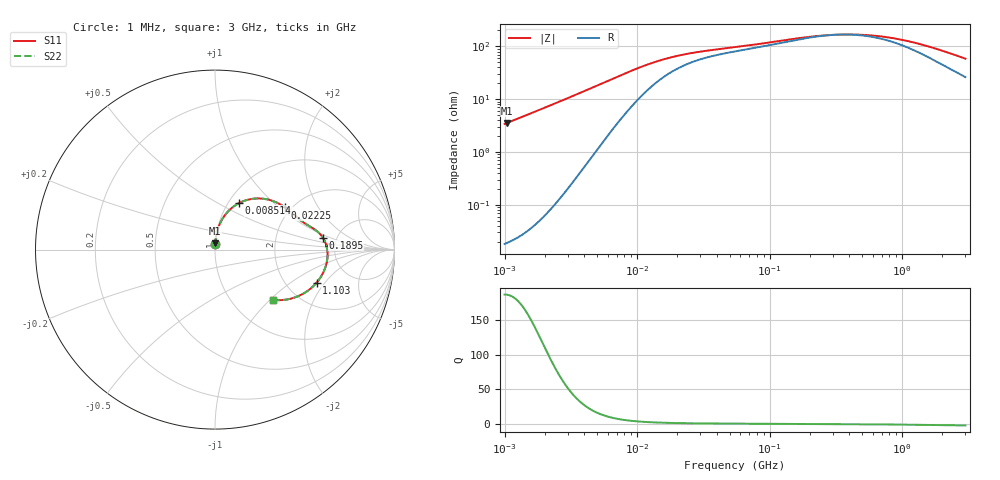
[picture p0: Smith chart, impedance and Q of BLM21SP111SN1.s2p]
! BLM21SP111SN1
# Hz S RI R 50
!Freq.(Hz) S11(Real) S11(Imag) S21(Real) S21(Imag) S12(Real) S12(Imag) S22(Real) S22(Imag)
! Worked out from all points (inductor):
!   401 points, 1 MHz to 3 GHz, reference 50 ohm
!   read as one part in series: L = 543 nH near 1.041 MHz
!   highest Q = 187 at 1.041 MHz (marker M1), where L = 541 nH
!   self-resonance near 332.2 MHz
!   S11 on the Smith chart (normalised r, x): 1 MHz: 1.00, +0.07; 8.514 MHz: 1.12, +0.64; 22.25 MHz: 1.86, +1.10; 189.5 MHz: 3.87, +0.81; 1.103 GHz: 2.90, -1.66; 3 GHz: 1.53, -1.05
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1000000  0.00134 0.0339  0.9987 -0.0339  0.9987 -0.0339  0.00134 0.0339
1040844  0.00144 0.0353  0.9986 -0.0353  0.9986 -0.0353  0.00144 0.0353
2139570  0.00613 0.0732  0.9939 -0.0732  0.9939 -0.0732  0.00613 0.0732
3823119  0.0223 0.1322  0.9777 -0.1322  0.9777 -0.1322  0.0223 0.1322
5938264  0.0625 0.2012  0.9375 -0.2012  0.9375 -0.2012  0.0625 0.2012
8513927  0.1352 0.2598  0.8648 -0.2598  0.8648 -0.2598  0.1352 0.2598
1.126754e7  0.2167 0.2838  0.7833 -0.2838  0.7833 -0.2838  0.2167 0.2838
1.461624e7  0.295 0.2788  0.705 -0.2788  0.705 -0.2788  0.295 0.2788
2.225279e7  0.3909 0.2352  0.6091 -0.2352  0.6091 -0.2352  0.3909 0.2352
3.190472e7  0.4408 0.1944  0.5592 -0.1944  0.5592 -0.1944  0.4408 0.1944
5.477226e7  0.491 0.1525  0.509 -0.1525  0.509 -0.1525  0.491 0.1525
1.148668e8  0.5587 0.1104  0.4413 -0.1104  0.4413 -0.1104  0.5587 0.1104
1.894586e8  0.6007 0.0666  0.3993 -0.0666  0.3993 -0.0666  0.6007 0.0666
2.094008e8  0.6072 0.0559  0.3928 -0.0559  0.3928 -0.0559  0.6072 0.0559
3.002264e8  0.6232 0.013  0.3768 -0.013  0.3768 -0.013  0.6232 0.013
4.219165e8  0.6273 -0.0322  0.3727 0.0322  0.3727 0.0322  0.6273 -0.0322
5.81181e8  0.6208 -0.079  0.3792 0.079  0.3792 0.079  0.6208 -0.079
8.005644e8  0.6018 -0.1304  0.3982 0.1304  0.3982 0.1304  0.6018 -0.1304
1.10276e9  0.5656 -0.1847  0.4344 0.1847  0.4344 0.1847  0.5656 -0.1847
1.45942e9  0.5162 -0.23  0.4838 0.23  0.4838 0.23  0.5162 -0.23
1.931433e9  0.4494 -0.265  0.5506 0.265  0.5506 0.265  0.4494 -0.265
3e9  0.3242 -0.2803  0.6758 0.2803  0.6758 0.2803  0.3242 -0.2803
